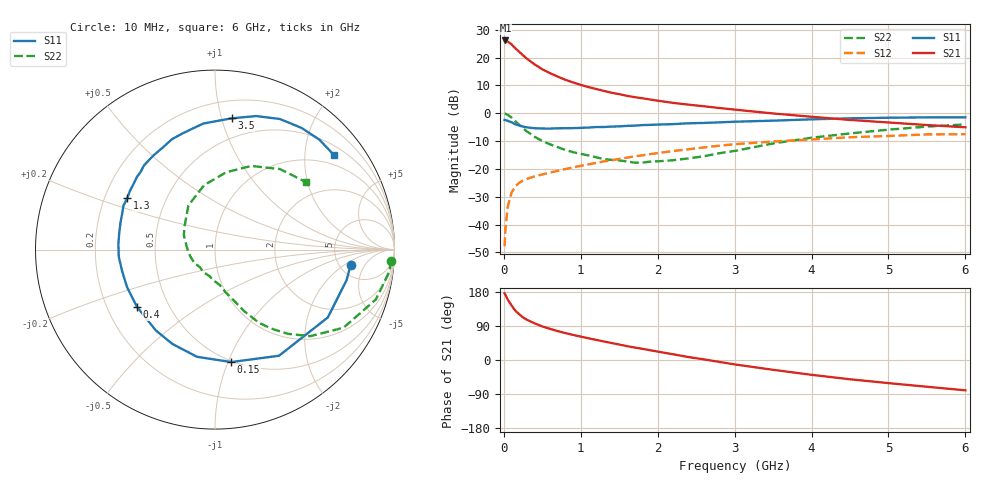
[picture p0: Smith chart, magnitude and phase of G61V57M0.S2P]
! SIEMENS Small Signal Semiconductors
! BFG193
! Si NPN RF Bipolar Junction Transistor in SOT223
! VCE = 1.5 V  IC = 7 mA
! Common Emitter S-Parameters:  August  1996
# GHz  S  MA  R  50
!  f  S11  S21  S12  S22
! GHz  MAG  ANG  MAG  ANG  MAG  ANG  MAG  ANG
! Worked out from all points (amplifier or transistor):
!   36 points, 10 MHz to 6 GHz, reference 50 ohm
!   highest |S21| = 26.2 dB at 20 MHz (marker M1)
!   |S21| within 3 dB of that: start of sweep to 157.6 MHz
!   unconditionally stable (mu >= 1): 975.4 MHz to 2.816 GHz
!   at 250 MHz: K = 0.43, MSG = 22.5 dB, |S12| = -24.1 dB
!   at 1.4 GHz: K = 1.09, MAG = 10.3 dB, |S12| = -16.9 dB
!   at 6 GHz: K = 0.93, MSG = 1.2 dB, |S12| = -7.5 dB
!   S11 on the Smith chart (normalised r, x): 10 MHz: 6.27, -2.56; 150 MHz: 0.49, -1.03; 400 MHz: 0.33, -0.30; 1.3 GHz: 0.30, +0.25; 3.5 GHz: 0.34, +1.08; 6 GHz: 0.72, +2.69
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0.01  0.7602 -6.5  20.34 175.7  0.0041 91.7  0.984 -3.6
0.02  0.7528 -13.0  20.34 172.4  0.0083 82.4  0.9787 -7.2
0.05  0.7336 -31.0  19.48 159.6  0.0206 74.7  0.9386 -17.2
0.1  0.6906 -58.9  17.3 144.1  0.0376 63.8  0.8379 -31.3
0.15  0.6331 -81.8  14.72 130.0  0.0488 54.5  0.7167 -42.3
0.2  0.6055 -99.6  12.73 120.6  0.0563 49.3  0.6209 -49.1
0.25  0.5766 -114.3  10.96 112.4  0.0621 45.5  0.5343 -55.0
0.3  0.5584 -126.1  9.563 106.2  0.0664 43.9  0.4733 -59.1
0.4  0.5391 -143.6  7.558 96.8  0.0736 41.6  0.3784 -64.7
0.5  0.5328 -157.0  6.175 88.6  0.0795 40.4  0.3172 -68.5
0.6  0.5313 -167.3  5.258 82.2  0.0861 40.6  0.277 -72.1
0.7  0.5376 -175.8  4.558 76.3  0.0926 40.7  0.2462 -75.8
0.9  0.5415 170.3  3.58 66.2  0.1069 40.9  0.2 -82.1
1.1  0.5544 159.1  2.956 57.3  0.1209 40.5  0.1748 -91.8
1.3  0.5667 149.7  2.524 48.9  0.1366 39.2  0.1505 -101.8
1.7  0.5995 133.7  1.951 32.9  0.168 35.4  0.1298 -128.3
2.2  0.6388 117.1  1.539 15.1  0.2097 27.3  0.1434 -165.5
2.8  0.6868 100.2  1.245 -5.0  0.2617 16.2  0.1915 154.9
3.5  0.7372 82.8  0.993 -25.9  0.3109 0.2  0.2871 121.1
4.5  0.8124 63.6  0.759 -50.9  0.3713 -19.3  0.4346 81.9
5.5  0.8447 46.5  0.615 -70.6  0.4172 -43.0  0.5763 51.1
6  0.8467 38.5  0.56 -80.0  0.4207 -56.6  0.6305 36.7
